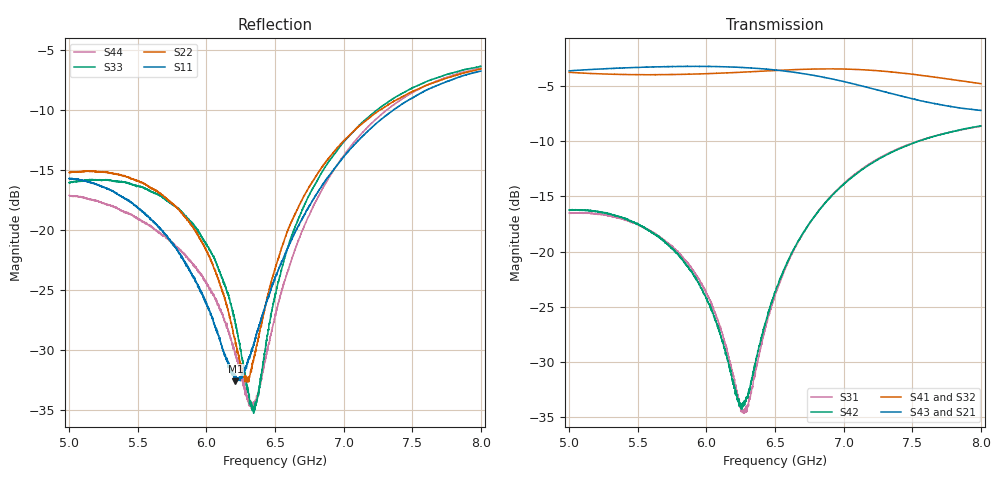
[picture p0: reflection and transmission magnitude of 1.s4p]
!Keysight Technologies,N5225A,MY51451420,A.10.40.12
!Date: Wednesday, May 11, 2016 10:11:01
!Correction: S11(Full 4 Port(1,2,3,4))
!S12(Full 4 Port(1,2,3,4))
!S13(Full 4 Port(1,2,3,4))
!S14(Full 4 Port(1,2,3,4))
!S21(Full 4 Port(1,2,3,4))
!S22(Full 4 Port(1,2,3,4))
!S23(Full 4 Port(1,2,3,4))
!S24(Full 4 Port(1,2,3,4))
!S31(Full 4 Port(1,2,3,4))
!S32(Full 4 Port(1,2,3,4))
!S33(Full 4 Port(1,2,3,4))
!S34(Full 4 Port(1,2,3,4))
!S41(Full 4 Port(1,2,3,4))
!S42(Full 4 Port(1,2,3,4))
!S43(Full 4 Port(1,2,3,4))
!S44(Full 4 Port(1,2,3,4))
!S4P File: Measurements: <S11,S12,S13,S14>,
!<S21,S22,S23,S24>,
!<S31,S32,S33,S34>,
!<S41,S42,S43,S44>:
# Hz S  dB  R 50
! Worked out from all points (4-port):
!   3201 points, 5 GHz to 8 GHz, reference 50 ohm
!   strongest paths, dB at 5 GHz, 5.75 GHz, 6.5 GHz, 7.25 GHz, 8 GHz:
!     S43: -3.6, -3.2, -3.5, -5.3, -7.2
!     S21: -3.7, -3.2, -3.6, -5.3, -7.0
!     S41: -3.7, -3.9, -3.6, -3.6, -4.8
!     S32: -3.7, -4.0, -3.6, -3.7, -4.8
!     S42: -16.2, -19.7, -23.7, -11.6, -8.6
!     S31: -16.5, -19.5, -24.0, -11.6, -8.6
!   lowest |S11| = -32.6 dB at 6.211 GHz (marker M1), VSWR 1.05, Z = 49.6 + j2.32 ohm
!   |S11| at or under -10 dB: start of sweep to 7.36 GHz
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5e9  -15.69 15.7  -3.66 105.0  -16.51 168.2  -3.72 10.2
     -3.66 104.9  -15.19 -109.6  -3.75 128.2  -16.24 -74.1
     -16.50 168.2  -3.75 128.3  -16.04 -133.2  -3.58 -143.7
     -3.72 10.2  -16.23 -74.1  -3.59 -143.7  -17.09 -131.5
5.664688e9  -19.87 -97.3  -3.24 11.7  -18.71 86.8  -3.93 -82.9
            -3.24 11.7  -16.96 163.0  -4.02 51.6  -18.77 -141.3
            -18.70 86.9  -4.02 51.6  -17.08 150.0  -3.22 137.6
            -3.94 -83.0  -18.80 -141.3  -3.22 137.6  -20.26 153.0
6.21125e9  -32.57 97.6  -3.28 -66.3  -32.16 49.9  -3.74 -160.7
           -3.28 -66.3  -29.34 56.9  -3.73 -13.1  -32.77 -158.3
           -32.23 48.9  -3.74 -13.2  -27.74 110.5  -3.25 72.0
           -3.75 -160.6  -32.90 -158.3  -3.25 72.1  -30.41 124.6
6.35375e9  -29.14 15.1  -3.39 -86.8  -31.27 116.1  -3.65 178.7
           -3.39 -86.8  -30.45 -44.6  -3.64 -30.6  -30.24 -93.9
           -31.27 116.2  -3.65 -30.6  -34.96 170.0  -3.35 54.7
           -3.65 178.6  -30.32 -94.5  -3.35 54.7  -34.45 175.0
6.978125e9  -14.19 -140.9  -4.54 -175.1  -14.10 57.0  -3.42 84.7
            -4.54 -175.1  -12.82 -174.4  -3.52 -109.9  -14.17 -139.3
            -14.09 57.0  -3.51 -110.0  -12.97 173.5  -4.49 -20.3
            -3.42 84.7  -14.16 -139.2  -4.50 -20.3  -14.12 175.0
7.475938e9  -9.13 127.1  -5.91 119.8  -10.28 -15.7  -3.85 8.5
            -5.91 119.8  -8.57 120.8  -3.99 -173.8  -10.30 160.6
            -10.27 -15.7  -3.98 -173.7  -8.28 116.0  -6.04 -74.1
            -3.85 8.4  -10.30 160.5  -6.05 -74.2  -8.68 115.4
8e9  -6.74 41.2  -7.00 56.5  -8.62 -87.9  -4.76 -69.0
     -6.99 56.4  -6.55 60.4  -4.83 121.5  -8.58 100.8
     -8.61 -87.8  -4.83 121.5  -6.33 55.1  -7.18 -124.1
     -4.75 -69.0  -8.59 100.8  -7.18 -124.1  -6.50 53.3
